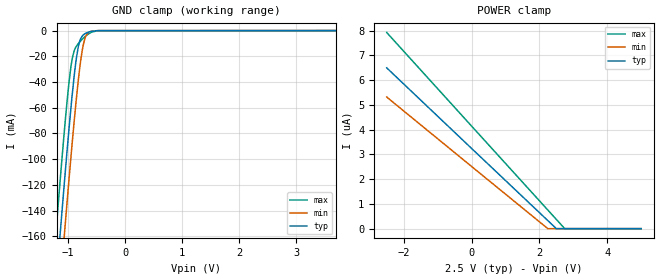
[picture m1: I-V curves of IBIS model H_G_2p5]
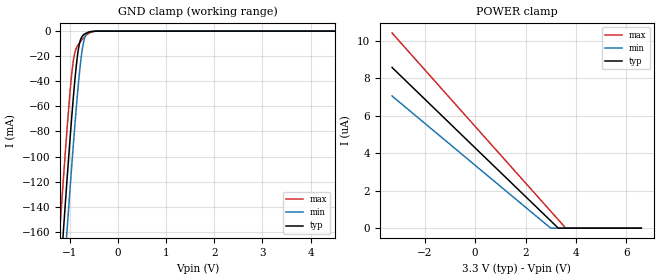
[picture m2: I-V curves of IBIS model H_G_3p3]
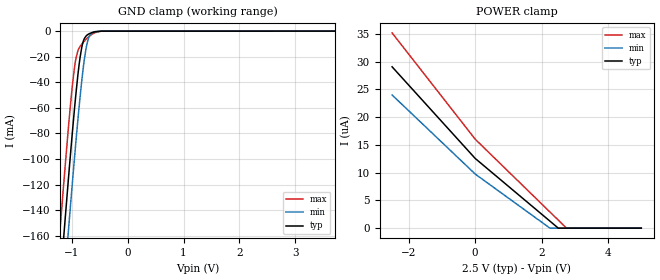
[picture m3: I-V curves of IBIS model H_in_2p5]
| Texas Instruments Incorporated
| 3.3V  LVCMOS High-Performance Clock Buffer
| Signal Rate: 200 kbps
| Marketing part#   Voltage Range   Package-type   #pins/pkg drawing
| cdclvc1108   2.25V - 3.6V   PW   16-pin TSSOP
[IBIS Ver]   4.1
[File name]   cdclvc1108.ibs
[File Rev]   1.0
[Date]   10/26/2010
[Source]   Model built from TISPICE simulations at:
   Texas Instruments Incorporated.
   Analog-eLab, HPA
   12500 TI Blvd
   Dallas, TX -75243
   For Support e-mail: elab_scm_ibis@list.ti.com
[Notes]   Revision History
   Rev 1.0: 08/02/2010
   - Model based on simulations from TIspiceD
   - C_comp values were obtained at 250MHz
   - For all buffers, Ccomp was obtained with the following corners:
   max C_comp was obtained at corner high VCC, low  temperature,
   strong process
   min C_comp was obtained at corner low  VCC, high temperature,
   weak process
   Rev 2.0: 10/26/2010
   - Appl. Eng. requested corrections for Vinh & Vinl
   In H_in_2p5 Vinh should be 1.65V.
   In H_in_3p3 Vinl should be 1.05V.
[Disclaimer] This product is designed as an aid for customers of Texas
   Instruments.
   No warranties, either expressed or implied, with respect
   to this third party software (if any) or with respect to
   its fitness for any particular purpose is claimed by Texas
   Instruments or the author. The software (if any) is provided
   solely on an "as is" basis. The entire risk as to its quality
   and performance is with the customer
[Copyright]   (C)Copyright 2010 Texas Instruments Incorporated.
   All rights reserved.
|   Component cvclvc1108pw
[Component]   cdclvc1108
[Manufacturer]  Texas Instruments Incorporated
[Package]   |16-pin TSSOP package
|   typ   min   max
R_pkg   0.19541   0.10694   0.23615
L_pkg   3.24219nH   2.54741nH   3.66684nH
C_pkg   0.48883pF   0.44642pF   0.52683pF
[Pin] signal_name   model_name   R_pin   L_pin   C_pin
1   CLKIN   H_in   0.17967 3.55170nH 0.52548pF
2   1G   H_G   0.20494 3.28620nH 0.50433pF
3   Y0   H_out   0.19948 3.01218nH 0.44642pF
4   GND   GND   0.1896  2.90713nH 0.45178pF
5   VDD   POWER   0.19534 2.96676nH 0.45537pF
6   Y4   H_out   0.21797 3.20523nH 0.45895pF
7   GND   GND   0.23615 3.61442nH 0.51896pF
8   Y6   H_out   0.17825 3.54517nH 0.52013pF
9   Y7   H_out   0.19043 3.66684nH 0.52683pF
10   VDD   POWER   0.23609 3.61160nH 0.52046pF
11   Y5   H_out   0.21797 3.20518nH 0.45680pF
12   GND   GND   0.19899 3.00421nH 0.45731pF
13   Y2   H_out   0.18960 2.90718nH 0.45532pF
14   VDD   POWER   0.10694 2.54741nH 0.49143pF
15   Y3   H_out   0.20526 3.28942nH 0.50603pF
16   Y1   H_out   0.17989 3.55435nH 0.52564pF
[Pin Mapping]pulldown_ref pullup_ref gnd_clamp_ref power_clamp_ref |ext_ref
 1   NC   NC   GNDBUS   PWRBUS   | CLKIN
 2   NC   NC   GNDBUS   PWRBUS   | 1G
 3   GNDBUS   PWRBUS   NC   NC   | Y0
 4   GNDBUS   NC   | GND
 5   NC   PWRBUS   | VDD
 6   GNDBUS   PWRBUS   NC   NC   | Y4
 7   GNDBUS   NC   | GND
 8   GNDBUS   PWRBUS   NC   NC   | Y6
 9   GNDBUS   PWRBUS   NC   NC   | Y7
10   NC   PWRBUS   | VDD
11   GNDBUS   PWRBUS   NC   NC   | Y5
12   GNDBUS   NC   | GND
13   GNDBUS   PWRBUS   NC   NC   | Y2
14   NC   PWRBUS   | VDD
15   GNDBUS   PWRBUS   NC   NC   | Y3
16   GNDBUS   PWRBUS   NC   NC   | Y1
[Model Selector] H_G
H_G_2p5   H_G Input model  at 2.5V
H_G_3p3   H_G Input model  at 3.3V
[Model Selector] H_in
H_in_2p5   H_in Input model at 2.5V
H_in_3p3   H_in Input model at 3.3V
[Model Selector] H_out
H_out_2p5   H_out Output model at 2.5V
H_out_3p3   H_out Output model at 3.3V
| Models and submodels in the file (6): H_G_2p5 (Input), H_G_3p3 (Input), H_in_2p5 (Input), H_in_3p3 (Input), H_out_2p5 (Output), H_out_3p3 (Output)
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|   H_G_2p5
[Model]   H_G_2p5
|Signal:   1G
Model_type   Input
Vinl   = 0.85
Vinh   = 1.65
|   typ   min   max
C_comp   910fF   809fF   967fF
[Voltage Range]   2.5   2.25   2.75
[Temperature Range]   25   85   -40
[Power Clamp Reference]   2.5   2.25   2.75
[GND Clamp Reference]   0   0   0
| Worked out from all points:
|   GND clamp passes 1 mA (typ) near -0.62 V on its own axis
[GND Clamp]
|   Voltage   I(typ)   I(min)   I(max)
-2.5V     -968.1mA   -1.007A    -929mA
-1.21V    -199mA     -240.4mA   -156.9mA
-1.15V    -165.5mA   -206.8mA   -123.9mA
-1.12V    -149.1mA   -190.2mA   -107.7mA
-1.064V   -118.8mA   -159.4mA   -78.45mA
-1.045V   -108.9mA   -149.3mA   -69.13mA
-947.5mV  -60.05mA   -98.34mA   -28.07mA
-850mV    -20.81mA   -51.87mA   -12.03mA
-771.2mV  -5.755mA   -21.65mA   -7.739mA
-681.3mV  -1.974mA   -3.841mA   -3.953mA
-463.7mV  -54uA      -32.29uA   -94.42uA
5V        0A         0A         0A
[POWER Clamp]
|   Voltage   I(typ)   I(min)   I(max)
-2.5V     6.5uA      5.321uA    7.929uA
2.251V    325.7nA    0A         752.1nA
2.502V    0A         0A         373.2nA
2.75V     0A         0A         0A
5V        0A         0A         0A
|   H_G_3p3
[Model]   H_G_3p3
|Signal:   1G
Model_type   Input
Vinl   = 1.05
Vinh   = 2.25
|   typ   min   max
C_comp   831.2f   785f   940.5f
[Voltage Range]   3.3   3   3.6
[Temperature Range]   25   85   -40
[Power Clamp Reference]   3.3   3   3.6
[GND Clamp Reference]   0   0   0
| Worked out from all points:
|   GND clamp passes 1 mA (typ) near -0.62 V on its own axis
[GND Clamp]
|   Voltage   I(typ)   I(min)   I(max)
-3.3V     -1.461A    -1.498A    -1.424A
-1.221V   -205.1mA   -246.6mA   -163.1mA
-1.206V   -196.8mA   -238.2mA   -154.8mA
-1.137V   -158.3mA   -199.5mA   -116.7mA
-1.063V   -118.2mA   -158.8mA   -77.87mA
-993.3mV  -82.31mA   -121.9mA   -45.27mA
-933.9mV  -53.76mA   -91.51mA   -24.11mA
-834.9mV  -16.5mA    -45.37mA   -11.07mA
-790.3mV  -7.806mA   -28.02mA   -8.666mA
-730.9mV  -3.374mA   -11.05mA   -5.922mA
-632mV    -1.127mA   -1.236mA   -2.355mA
6.6V      0A         0A         0A
[POWER Clamp]
|   Voltage   I(typ)   I(min)   I(max)
-3.3V     8.58uA     7.058uA    10.42uA
3.001V    391.5nA    0A         903.2nA
3.303V    0A         0A         447.8nA
3.6V      0A         0A         0A
6.6V      0A         0A         0A
|   H_in_2p5
[Model]   H_in_2p5
|Signal:   CLK_IN
Model_type   Input
Vinl   = 0.85
Vinh   = 1.65
|   typ   min   max
C_comp   0.943pF   0.765pF   1.207pF
[Voltage Range]   2.5   2.25   2.75
[Temperature Range]   25   85   -40
[Power Clamp Reference]   2.5   2.25   2.75
[GND Clamp Reference]   0   0   0
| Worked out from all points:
|   GND clamp passes 1 mA (typ) near -0.62 V on its own axis
[GND Clamp]
|   Voltage   I(typ)   I(min)   I(max)
-2.5V     -968.1mA   -1.007A    -929mA
-1.21V    -199mA     -240.4mA   -156.9mA
-1.15V    -165.6mA   -206.8mA   -123.9mA
-1.12V    -149.1mA   -190.2mA   -107.7mA
-1.064V   -118.8mA   -159.4mA   -78.47mA
-1.045V   -108.9mA   -149.3mA   -69.14mA
-947.5mV  -60.06mA   -98.34mA   -28.08mA
-850mV    -20.82mA   -51.87mA   -12.04mA
-771.2mV  -5.763mA   -21.66mA   -7.749mA
-681.3mV  -1.981mA   -3.847mA   -3.963mA
-463.7mV  -60.38uA   -37.46uA   -102.3uA
5V        0A         0A         0A
[POWER Clamp]
|   Voltage   I(typ)   I(min)   I(max)
-2.5V     29.05uA    23.98uA    35.15uA
1.25mV    12.55uA    9.742uA    16.01uA
2.251V    1.261uA    0A         2.905uA
2.502V    0A         0A         1.442uA
2.75V     0A         0A         0A
5V        0A         0A         0A
